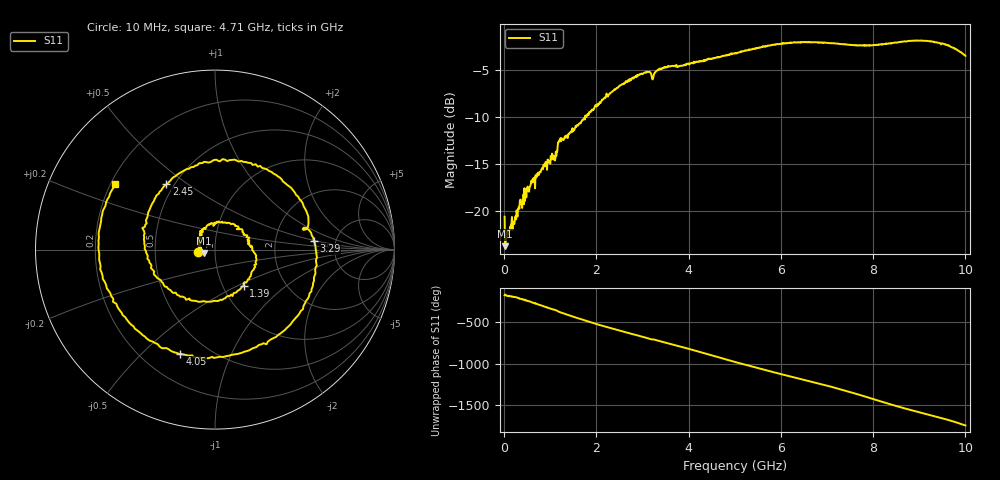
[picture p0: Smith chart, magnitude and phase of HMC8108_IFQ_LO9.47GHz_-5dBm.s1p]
! Analog Devices, Inc.
! 1 Analog Way
! Wilmington, MA 01887
! http://www.analog.com
! Date:  2021-09-07 NN
! Board Name:  EV1HMC8108LC5 Revision A with HMC8108LC5 installed
! File Description:  S-Parameters for evaluation board without connectors or board loss de-embedded
! File Generation:  Calibrated Network Analyzer
! Chip Part Number:  HMC8108
! Chip Description:  X-Band, GaAs, MMIC, Low Noise Converter
! Chip Frequency:  9 to 10 GHz
! Chip Package:  LCC, 5 x 5 x 1.12 mm
! Chip State:
!  Temperature:  25C
!  LO Frequency:  9.47GHz
!  LO Power:  -5dBm
! Note:
!  Analog Devices supplies this data as a sample of measured data at the evaluation board
!  ports for this product.  Your particular data for this product may vary.
!  Analog Devices reserves the right to change this data at anytime.
!  All lines below in this file are as is from the Network Analyzer.
!Keysight Technologies,N5245A,MY49151104,A.10.65.16
!Date: Thursday, August 19, 2021 13:44:53
!Correction: S22(Full 2 Port(1,2))
!S1P File: Measurement: S22:
# Hz S  dB  R 50
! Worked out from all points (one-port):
!   1000 points, 10 MHz to 10 GHz, reference 50 ohm
!   lowest |S11| = -23.7 dB at 20 MHz (marker M1), VSWR 1.14, Z = 44.1 - j1.61 ohm
!   |S11| at or under -10 dB: start of sweep to 1.756 GHz
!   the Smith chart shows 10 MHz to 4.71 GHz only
!   S11 on the Smith chart (normalised r, x): 10 MHz: 0.83, -0.02; 1.39 GHz: 1.25, -0.54; 2.45 GHz: 0.45, +0.42; 3.29 GHz: 3.40, +0.48; 4.05 GHz: 0.35, -0.66; 4.71 GHz: 0.22, +0.28
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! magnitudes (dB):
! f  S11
! 10 MHz  -20.6
! 20 MHz  -23.7
! 70 MHz  -22.0
! 120 MHz  -22.1
! 230 MHz  -21.0
! 320 MHz  -19.5
! 610 MHz  -16.7
! 900 MHz  -14.8
! 1.1 GHz  -14.6
! 1.21 GHz  -12.5
! 1.26 GHz  -12.3
! 1.39 GHz  -11.8
! 2.17 GHz  -8.0
! 2.45 GHz  -6.9
! 2.51 GHz  -6.7
! 2.94 GHz  -5.4
! 3.12 GHz  -5.2
! 3.23 GHz  -5.8
! 3.29 GHz  -5.1
! 3.76 GHz  -4.7
! 4.05 GHz  -4.2
! 4.71 GHz  -3.5
! 5.01 GHz  -3.2
! 6.26 GHz  -2.1
! 7.51 GHz  -2.3
! 8.76 GHz  -1.9
! 9.53 GHz  -2.2
! 10 GHz  -3.5
